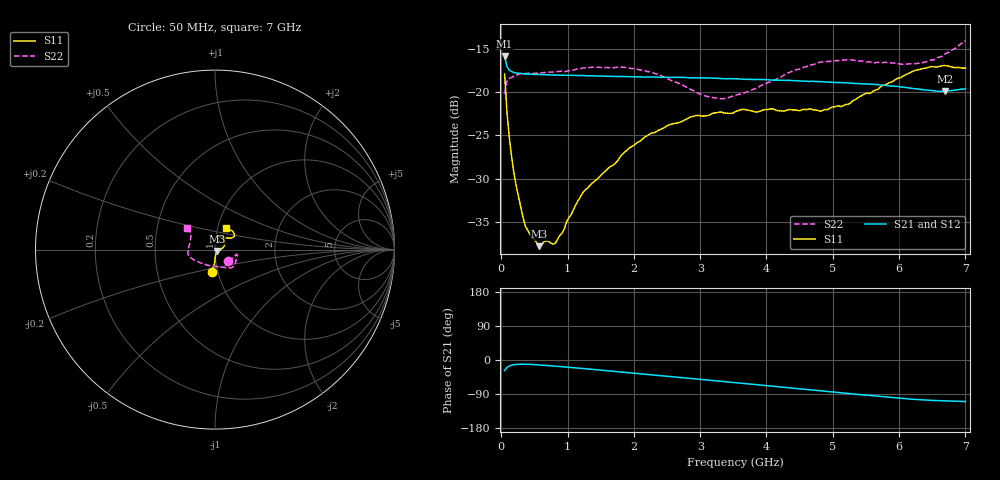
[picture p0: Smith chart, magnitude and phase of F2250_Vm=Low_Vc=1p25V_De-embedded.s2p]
! Integrated Device Technology
! Corporate Headquarters
! 6024 Silver Creek Valley Road
! San Jose, CA 95138  USA
! Phone:  1-408-284-8200
! Toll Free:  1-800-223-1366
! Webpage:  http://www.idt.com/
! Timing and RF Division
! 515 Groton Road, Suite 102
! Westford, MA 01886-6024
! Device:  F2250
! Description: Voltage Variable RF Attenuator
! Frequency:  50.0 -  6000.00 MHz
! Package:  3x3 mm Thin QFN Plastic Package: 16 pin
! Ports:  2 RF, 3 DC
!  Pin  1  = GND
!  Pin  2  = NC
!  Pin  3  = RF1  = Port 1
!  Pin  4  = NC
!  Pin  5  = GND
!  Pin  6  = GND
!  Pin  7  = GND
!  Pin  8  = GND
!  Pin  9  = NC
!  Pin 10  = RF2  = Port 2
!  Pin 11  = NC
!  Pin 12  = GND
!  Pin 13  = GND
!  Pin 14  = VCNTRL
!  Pin 15  = VDD
!  Pin 16  = VMODE
! Vcntrl:  1.250 Volts
! Vmode:  +0.000 Volts
! Vdd:  +3.30  Volts
! Current:  1.193 mA
! Data:  The device was measured on a the F2250 evaluation board which has
!  individual transmission lines to the RF pins.  Data was collected
!  using a calibrated network analyzer.  The evaluation board was
!  de-embedded using a TRL calibration technique.
!  The reference plane is the edge of the package pin.
! Misc:  SN 10
!  Action Tracker AT0258
! Date Measured:  2014-11-26
! Date:  2015-10-15  MJV
! Note:
!  Integrated Device Technology supplies this data as a sample of measured
!  data at the package pin for this product.  Your particular data for this
!  product may vary.
!  Data was taken at 25 degrees C.
!  Integrated Device Technology reserves the right to change this data at anytime.
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# GHz S dB R 50
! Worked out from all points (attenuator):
!   201 points, 50 MHz to 7 GHz, reference 50 ohm
!   highest |S21| = -15.84 dB at 50 MHz (marker M1); lowest = -19.9 dB at 6.687 GHz (marker M2)
!   lowest |S11| = -37.8 dB at 571.2 MHz (marker M3), VSWR 1.03, Z = 51 - j0.829 ohm
!   |S11| at or under -10 dB: start of sweep to end of sweep
!   |S22| runs from -20.8 to -14.1 dB; largest |S21 - S12| = 0.00065
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0.05  -17.94 -98.7  -15.84 -27.7  -15.86 -27.7  -20.22 -40.9
0.08475  -22.24 -91.6  -17.06 -19.8  -17.07 -19.8  -18.75 -19.8
0.1195  -25.16 -90.0  -17.48 -15.8  -17.47 -15.8  -18.46 -14.3
0.189  -29.31 -85.1  -17.76 -12.4  -17.75 -12.3  -18.17 -12.1
0.22375  -30.79 -80.6  -17.81 -11.6  -17.82 -11.6  -18.08 -12.3
0.36275  -35.45 -67.5  -17.93 -11.2  -17.93 -11.2  -17.88 -13.1
0.57125  -37.79 -39.0  -17.98 -13.1  -17.99 -13.1  -17.84 -18.1
0.6755  -37.17 -34.0  -18.01 -14.4  -18.00 -14.4  -17.74 -20.8
0.8145  -37.45 -20.5  -18.06 -16.2  -18.06 -16.2  -17.68 -24.7
1.2315  -31.60 -5.9  -18.10 -22.4  -18.12 -22.4  -17.23 -34.3
1.9265  -26.48 15.4  -18.23 -33.4  -18.21 -33.4  -17.24 -45.8
2.37825  -24.39 26.8  -18.30 -40.7  -18.31 -40.7  -17.99 -54.4
2.86475  -22.86 42.0  -18.36 -48.7  -18.36 -48.7  -19.74 -71.3
3.07325  -22.76 48.7  -18.38 -52.2  -18.39 -52.2  -20.45 -82.7
3.3165  -22.32 57.1  -18.45 -56.3  -18.44 -56.3  -20.78 -99.2
3.525  -22.31 61.8  -18.48 -59.7  -18.50 -59.7  -20.39 -113.6
4.7065  -22.07 67.2  -18.77 -79.5  -18.76 -79.6  -16.84 -162.0
5.22775  -21.42 50.2  -18.95 -88.3  -18.95 -88.3  -16.30 -171.6
5.85325  -18.94 35.2  -19.30 -98.5  -19.31 -98.5  -16.66 174.8
6.33975  -17.34 37.5  -19.71 -105.2  -19.71 -105.3  -16.64 157.5
6.68725  -16.95 46.5  -19.94 -107.5  -19.92 -107.6  -15.64 145.2
7  -17.25 63.0  -19.62 -109.7  -19.61 -109.8  -14.06 142.9
